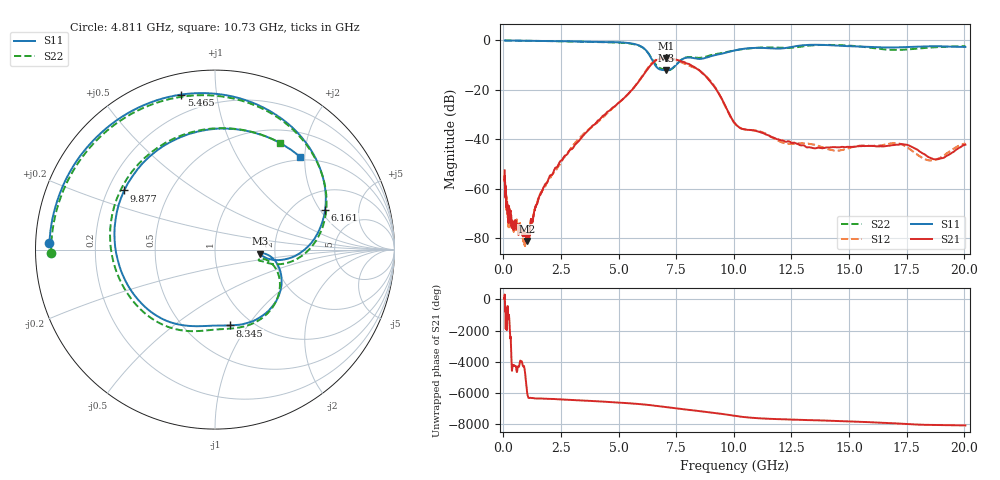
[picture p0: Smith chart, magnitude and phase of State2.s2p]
# Hz S DB R 50
!freq MagS11 AngS11 MagS21 AngS21 MagS12 AngS12 MagS22 AngS22
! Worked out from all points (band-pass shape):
!   1601 points, 50 MHz to 20.05 GHz, reference 50 ohm
!   highest |S21| = -7.12 dB at 7.076 GHz (marker M1); lowest = -81.1 dB at 1.013 GHz (marker M2)
!   |S21| within 3 dB of the highest: 6.375 GHz to 8.154 GHz (1.778 GHz wide, 24.5 % of centre)
!   lowest |S11| = -12.0 dB at 7.076 GHz (marker M3), VSWR 1.67, Z = 83.2 - j4.09 ohm
!   |S11| at or under -10 dB: 6.585 GHz to 7.474 GHz (888.5 MHz wide, 12.6 % of centre)
!   |S22| runs from -12.0 to 0.0 dB; largest |S21 - S12| = 0.029
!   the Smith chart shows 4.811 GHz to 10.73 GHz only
!   S11 on the Smith chart (normalised r, x): 4.811 GHz: 0.04, +0.02; 5.465 GHz: 0.10, +0.80; 6.161 GHz: 2.90, +2.23; 8.345 GHz: 0.80, -0.83; 9.877 GHz: 0.27, +0.28; 10.73 GHz: 0.93, +1.90
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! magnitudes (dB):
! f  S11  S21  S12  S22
! 50 MHz  0.0  -52.5  -56.9  0.0
! 135.9 MHz  0.0  -67.4  -66.4  0.0
! 159.7 MHz  0.0  -66.2  -64.7  0.0
! 222.9 MHz  0.0  -73.7  -74.6  0.0
! 244.8 MHz  0.0  -67.3  -70.8  0.0
! 369.6 MHz  0.0  -73.9  -74.3  0.0
! 586 MHz  -0.1  -75.2  -73.1  -0.1
! 1.005 GHz  -0.1  -80.6  -80.0  -0.1
! 1.013 GHz  -0.1  -81.1  -80.4  -0.1
! 2.722 GHz  -0.3  -46.3  -46.2  -0.4
! 4.811 GHz  -0.7  -26.8  -26.8  -0.8
! 5.465 GHz  -1.1  -21.1  -21.1  -1.2
! 6.161 GHz  -3.7  -12.8  -12.5  -3.8
! 7.076 GHz  -12.0  -7.1  -7.0  -12.0
! 7.402 GHz  -10.7  -7.5  -7.7  -10.8
! 8.345 GHz  -7.3  -11.1  -11.3  -7.0
! 9.877 GHz  -4.4  -31.1  -31.3  -4.3
! 10.73 GHz  -3.1  -36.2  -36.2  -3.1
! 14.31 GHz  -2.0  -43.1  -44.4  -1.8
! 17 GHz  -2.8  -42.2  -41.5  -3.8
! 18.53 GHz  -2.3  -47.5  -48.5  -2.9
! 20.05 GHz  -2.6  -42.1  -41.7  -2.3
